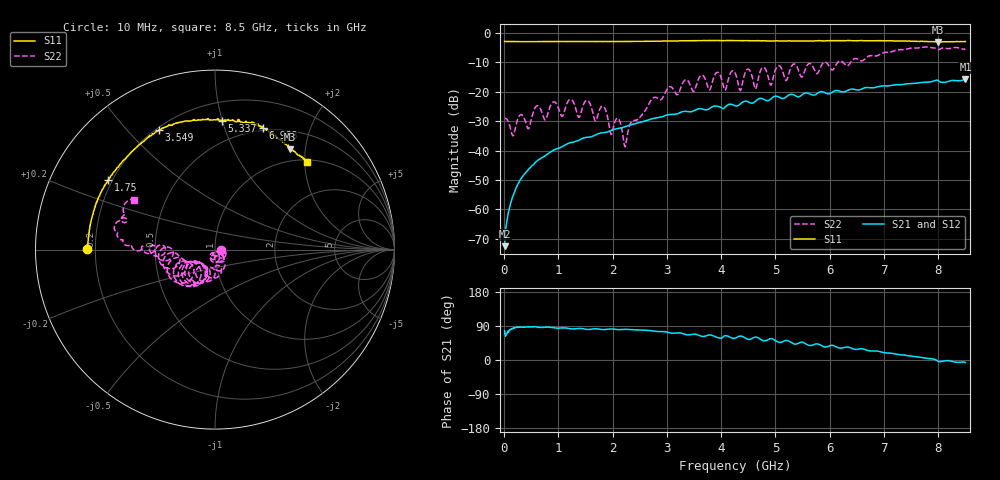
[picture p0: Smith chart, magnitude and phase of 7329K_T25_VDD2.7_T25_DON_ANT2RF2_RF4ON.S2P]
!Agilent Technologies,E5071C,MY46417908,A.11.23
!Date: Mon Aug 31 18:03:19 2020
!Data & Calibration Information:
!Freq	S11:SOLT2(ON)	S21:SOLT2(ON)	S12:SOLT2(ON)	S22:SOLT2(ON)
!PortZ  Port1:50+j0  Port2:50+j0
!Above PortZ is port z conversion or system Z0 setting when saving the data.
!When reading, reference impedance value at option line is always used.
# Hz S dB R 50
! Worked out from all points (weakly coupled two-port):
!   1601 points, 10 MHz to 8.5 GHz, reference 50 ohm
!   highest |S21| = -15.78 dB at 8.5 GHz (marker M1); lowest = -72.5 dB at 10 MHz (marker M2)
!   lowest |S11| = -3.1 dB at 8.001 GHz (marker M3), VSWR 5.60, Z = 39.4 + j85.7 ohm
!   |S11| at or under -10 dB: nowhere
!   |S22| runs from -38.7 to -4.8 dB; largest |S21 - S12| = 0.0018
!   S11 on the Smith chart (normalised r, x): 10 MHz: 0.17, +0.00; 1.75 GHz: 0.18, +0.29; 3.549 GHz: 0.21, +0.61; 5.337 GHz: 0.33, +1.00; 6.988 GHz: 0.47, +1.36; 8.5 GHz: 1.04, +2.05
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1e7  -2.94 179.8  -72.46 77.0  -72.64 74.4  -29.07 -2.1
1.426562e8  -2.98 176.9  -56.67 83.0  -56.64 82.2  -34.28 -10.4
3.602125e8  -3.00 172.5  -48.37 86.5  -48.33 86.7  -28.57 -6.6
1.219825e9  -2.97 156.3  -37.31 82.4  -37.32 82.4  -22.57 -62.7
1.426769e9  -2.97 152.9  -36.01 83.0  -36.01 82.9  -26.48 -62.8
1.75045e9  -2.97 147.0  -34.18 81.5  -34.16 81.5  -26.53 -84.6
1.845962e9  -2.97 145.1  -33.90 80.2  -33.89 80.2  -25.30 -115.1
1.973312e9  -2.96 143.0  -33.19 81.9  -33.19 81.9  -34.50 -107.4
2.105969e9  -2.95 140.3  -32.48 80.1  -32.48 80.1  -29.16 -101.2
2.233319e9  -2.96 137.9  -31.88 80.9  -31.89 80.9  -38.74 -72.6
2.843538e9  -2.84 126.2  -28.81 75.2  -28.81 75.2  -22.42 -63.5
3.549269e9  -2.67 115.2  -26.01 67.4  -26.00 67.4  -17.41 -89.8
4.255e9  -2.66 105.7  -24.77 57.5  -24.77 57.5  -13.59 -143.6
4.631744e9  -2.72 99.6  -23.29 60.5  -23.29 60.3  -19.12 -134.0
4.7644e9  -2.74 97.5  -22.41 51.5  -22.40 51.5  -11.77 -130.1
4.912975e9  -2.78 94.7  -22.51 56.3  -22.52 56.4  -17.79 -138.0
5.337475e9  -2.85 86.8  -21.09 42.5  -21.08 42.5  -10.59 -147.8
5.671769e9  -2.82 81.1  -21.10 38.7  -21.08 38.7  -10.95 -171.4
6.987719e9  -2.75 68.7  -18.03 19.8  -18.05 19.7  -6.78 179.3
7.088538e9  -2.76 66.5  -18.01 18.3  -18.04 18.0  -6.59 176.6
8.001212e9  -3.13 53.3  -16.28 -3.9  -16.31 -3.9  -5.74 161.8
8.5e9  -2.99 43.6  -15.78 -6.5  -15.83 -6.8  -5.53 148.2
